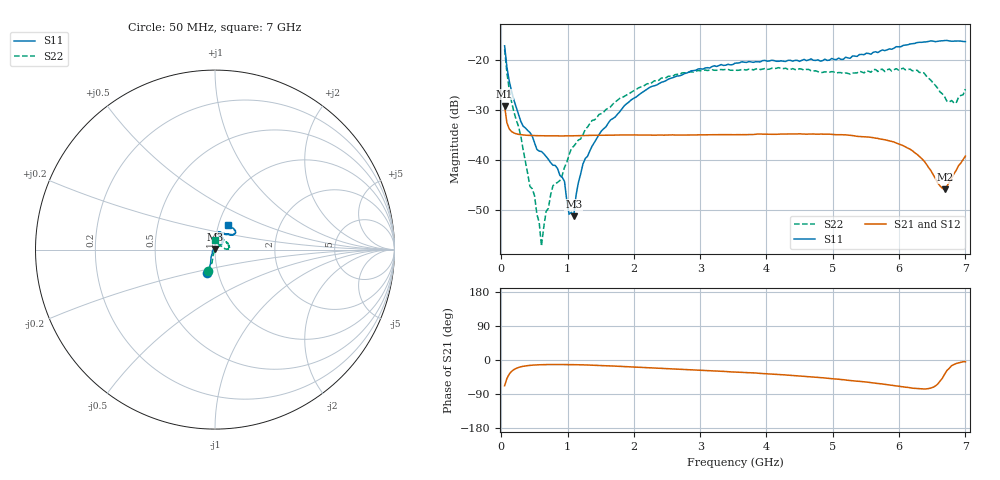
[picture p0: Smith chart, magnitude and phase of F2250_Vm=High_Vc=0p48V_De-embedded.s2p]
! Integrated Device Technology
! Corporate Headquarters
! 6024 Silver Creek Valley Road
! San Jose, CA 95138  USA
! Phone:  1-408-284-8200
! Toll Free:  1-800-223-1366
! Webpage:  http://www.idt.com/
! Timing and RF Division
! 515 Groton Road, Suite 102
! Westford, MA 01886-6024
! Device:  F2250
! Description: Voltage Variable RF Attenuator
! Frequency:  50.0 -  6000.00 MHz
! Package:  3x3 mm Thin QFN Plastic Package: 16 pin
! Ports:  2 RF, 3 DC
!  Pin  1  = GND
!  Pin  2  = NC
!  Pin  3  = RF1  = Port 1
!  Pin  4  = NC
!  Pin  5  = GND
!  Pin  6  = GND
!  Pin  7  = GND
!  Pin  8  = GND
!  Pin  9  = NC
!  Pin 10  = RF2  = Port 2
!  Pin 11  = NC
!  Pin 12  = GND
!  Pin 13  = GND
!  Pin 14  = VCNTRL
!  Pin 15  = VDD
!  Pin 16  = VMODE
! Vcntrl:  0.480 Volts
! Vmode:  +3.300 Volts
! Vdd:  +3.30  Volts
! Current:  1.268 mA
! Data:  The device was measured on a the F2250 evaluation board which has
!  individual transmission lines to the RF pins.  Data was collected
!  using a calibrated network analyzer.  The evaluation board was
!  de-embedded using a TRL calibration technique.
!  The reference plane is the edge of the package pin.
! Misc:  SN 10
!  Action Tracker AT0258
! Date Measured:  2014-11-26
! Date:  2015-10-15  MJV
! Note:
!  Integrated Device Technology supplies this data as a sample of measured
!  data at the package pin for this product.  Your particular data for this
!  product may vary.
!  Data was taken at 25 degrees C.
!  Integrated Device Technology reserves the right to change this data at anytime.
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# GHz S dB R 50
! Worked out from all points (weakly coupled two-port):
!   201 points, 50 MHz to 7 GHz, reference 50 ohm
!   highest |S21| = -29.25 dB at 50 MHz (marker M1); lowest = -46.0 dB at 6.687 GHz (marker M2)
!   lowest |S11| = -51.3 dB at 1.093 GHz (marker M3), VSWR 1.01, Z = 50 + j0.271 ohm
!   |S11| at or under -10 dB: start of sweep to end of sweep
!   |S22| runs from -57.3 to -17.9 dB; largest |S21 - S12| = 4.9e-05
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0.05  -17.17 -108.5  -29.25 -68.0  -29.25 -68.0  -17.87 -108.1
0.1195  -24.20 -111.9  -33.81 -37.3  -33.81 -37.2  -25.94 -104.9
0.29325  -32.28 -127.3  -34.98 -18.0  -34.98 -18.0  -35.17 -107.2
0.43225  -34.55 -145.2  -35.13 -14.1  -35.13 -14.1  -45.36 -132.9
0.50175  -36.62 -147.8  -35.16 -13.2  -35.16 -13.2  -47.23 -142.2
0.606  -38.36 -162.6  -35.20 -12.4  -35.19 -12.4  -57.32 155.1
0.6755  -39.34 -163.7  -35.21 -12.1  -35.21 -12.1  -50.37 88.5
0.77975  -41.10 176.5  -35.22 -11.9  -35.22 -11.9  -45.18 79.2
0.9535  -44.34 170.7  -35.23 -12.0  -35.23 -12.0  -41.52 67.4
1.023  -50.92 139.7  -35.22 -12.1  -35.22 -12.1  -38.96 56.0
1.0925  -51.33 88.7  -35.20 -12.3  -35.20 -12.3  -37.30 53.0
1.12725  -47.16 60.7  -35.19 -12.4  -35.19 -12.4  -36.71 48.3
1.2315  -40.86 40.5  -35.16 -12.8  -35.16 -12.8  -35.00 40.7
1.6485  -32.02 40.9  -35.08 -15.7  -35.08 -15.7  -29.39 41.7
2.37825  -24.75 46.6  -35.05 -21.7  -35.06 -21.7  -24.06 44.2
3.525  -20.66 71.7  -34.99 -31.6  -34.99 -31.6  -22.03 67.7
4.7065  -20.06 72.0  -34.84 -45.0  -34.85 -45.0  -22.21 67.2
5.85325  -17.79 40.5  -36.23 -65.8  -36.23 -65.9  -21.82 18.3
6.3745  -16.40 40.9  -40.22 -76.4  -40.24 -76.5  -22.60 2.0
6.68725  -16.12 47.8  -45.95 -37.3  -45.93 -36.9  -27.39 24.0
6.861  -16.22 54.5  -42.13 -9.2  -42.08 -9.3  -28.64 58.5
7  -16.33 62.4  -39.27 -4.5  -39.23 -4.6  -25.84 88.0
